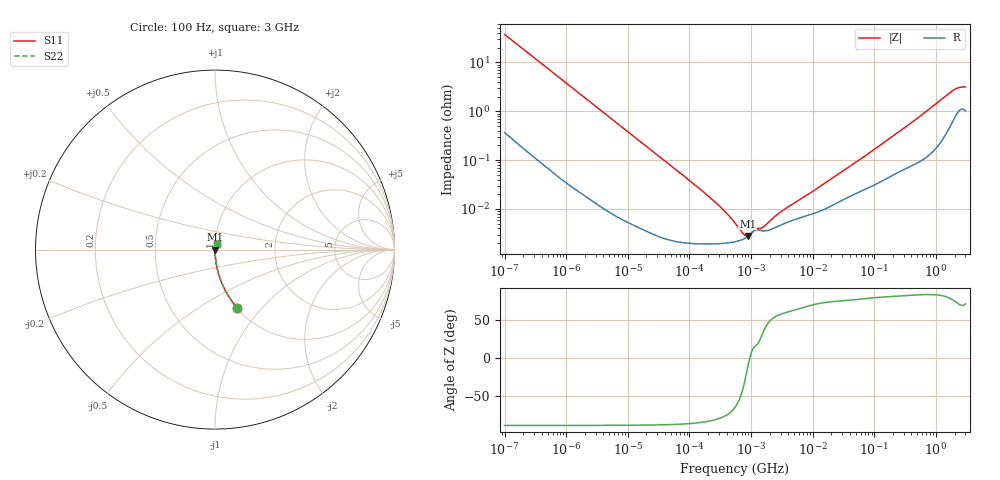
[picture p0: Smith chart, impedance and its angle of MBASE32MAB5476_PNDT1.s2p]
! MBASE32MAB5476_PNDT1  S-PARAMETER MODEL  ( Standard Model )
! Model Generated by TAIYO YUDEN Corporation (http://www.ty-top.com)
! Version 1.0
! TAIYO YUDEN Control No. 220601
! Copyright(c) 2016 TAIYO YUDEN CO.,LTD. All Rights Reserved.
! Product Description (link to TY-COMPAS)
! https://ds.yuden.co.jp/TYCOMPAS/or/detail?pn=MBASE32MAB5476KPNDT1&u=M
! Products Name : Multilayer Ceramic Capacitors
! Characteristics :
!  Capacitance : 47 [uF] , Rated Voltage : 16 [V] , TCC : X5R
!  Case Size : 3.2 x 2.5 / 0.126 x 0.098 [mm/inch] , Thickness : 2.5 / 0.098 [mm/inch]
!  (Conditions: Temperature = 25 [degC] , DC Bias Voltage = 0 [V])
! External Node Assignments :
!  1  o---| |---o  2
! GND o---------o GND
! Frequency Range : 100Hz  -  3GHz  [ 401 STEP ]
# MHZ S RI R 50
! Freq[MHz].  S11 Real  S11 Imag  S21 Real  S21 Imag  S12 Real  S12 Imag  S22 Real  S22 Imag
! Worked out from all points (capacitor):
!   401 points, 100 Hz to 3 GHz, reference 50 ohm
!   read as one part in series: C = 42.5 uF near 109 Hz
!   lowest |Z| = 2.79 mohm at 879.4 kHz (marker M1)
!   series resonance near 955.3 kHz, so ESL is about 650 pH
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0.0001  0.1249 -0.3258  0.8751 0.3258  0.8751 0.3258  0.1249 -0.3258
0.000114  0.0998 -0.2949  0.9002 0.2949  0.9002 0.2949  0.0998 -0.2949
0.000175  0.0456 -0.2041  0.9544 0.2041  0.9544 0.2041  0.0456 -0.2041
0.000348  0.0125 -0.1066  0.9875 0.1066  0.9875 0.1066  0.0125 -0.1066
0.000724  0.00318 -0.052  0.9968 0.052  0.9968 0.052  0.00318 -0.052
0.001788  0.000655 -0.0212  0.9993 0.0212  0.9993 0.0212  0.000655 -0.0212
0.031977  2.86e-05 -0.00121  1 0.00121  1 0.00121  2.86e-05 -0.00121
0.144239  1.95e-05 -0.000263  1 0.000263  1 0.000263  1.95e-05 -0.000263
0.326774  1.97e-05 -0.000105  1 0.000105  1 0.000105  1.97e-05 -0.000105
0.371814  1.99e-05 -8.83e-05  1 8.83e-05  1 8.83e-05  1.99e-05 -8.83e-05
0.547723  2.14e-05 -4.72e-05  1 4.72e-05  1 4.72e-05  2.14e-05 -4.72e-05
0.87939  2.72e-05 -6.26e-06  1 6.26e-06  1 6.26e-06  2.72e-05 -6.26e-06
3.486191  5.07e-05 8.48e-05  0.9999 -8.48e-05  0.9999 -8.48e-05  5.07e-05 8.48e-05
3.966702  5.42e-05 9.57e-05  0.9999 -9.57e-05  0.9999 -9.57e-05  5.42e-05 9.57e-05
9.794414  7.89e-05 0.000212  0.9999 -0.000212  0.9999 -0.000212  7.89e-05 0.000212
59.714  0.00023 0.00103  0.9998 -0.00103  0.9998 -0.00103  0.00023 0.00103
175.1444  0.000458 0.00272  0.9995 -0.00272  0.9995 -0.00272  0.000458 0.00272
492.0662  0.000917 0.00706  0.9991 -0.00706  0.9991 -0.00706  0.000917 0.00706
1789.813  0.00616 0.0246  0.9938 -0.0246  0.9938 -0.0246  0.00616 0.0246
2036.508  0.00831 0.0269  0.9917 -0.0269  0.9917 -0.0269  0.00831 0.0269
2317.205  0.0106 0.0282  0.9894 -0.0282  0.9894 -0.0282  0.0106 0.0282
3000  0.011 0.0293  0.989 -0.0293  0.989 -0.0293  0.011 0.0293
